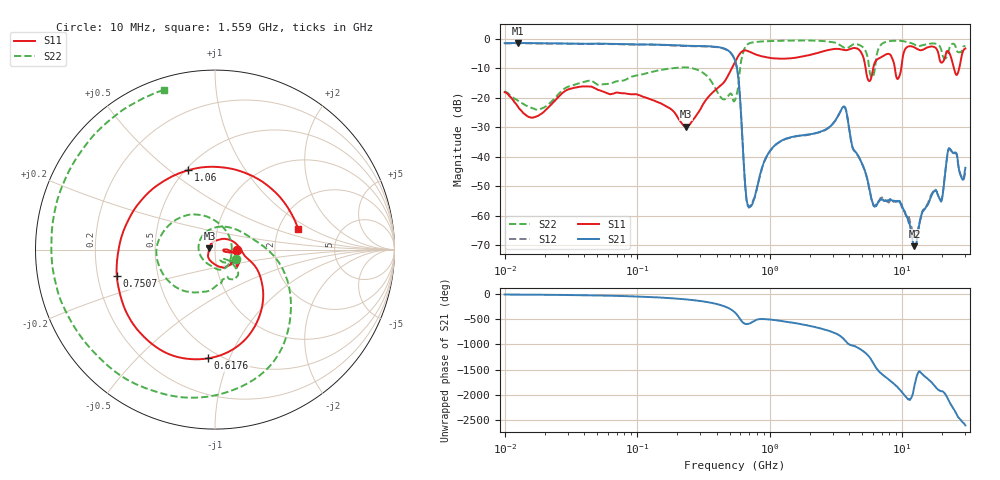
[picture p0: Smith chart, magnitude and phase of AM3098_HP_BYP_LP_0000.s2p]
!Agilent Technologies,E8364B,MY43040894,A.07.50.67
!Agilent E8364B: A.07.50.67
!Date: Wednesday, June 17, 2020 09:18:11
!Correction: S11(Full 2 Port(1,2))
!S21(Full 2 Port(1,2))
!S12(Full 2 Port(1,2))
!S22(Full 2 Port(1,2))
!S2P File: Measurements: S11, S21, S12, S22:Log Frequency Sweep
# Hz S  dB  R 50
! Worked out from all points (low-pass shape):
!   1601 points, 10 MHz to 30 GHz, reference 50 ohm
!   highest |S21| = -1.43 dB at 12.59 MHz (marker M1); lowest = -70.3 dB at 12.37 GHz (marker M2)
!   |S21| within 3 dB of the highest: start of sweep to 500.4 MHz
!   lowest |S11| = -29.8 dB at 235.1 MHz (marker M3), VSWR 1.07, Z = 47 + j0.748 ohm
!   |S11| at or under -10 dB: 5.299 GHz to 6.04 GHz (741.2 MHz wide, 13.1 % of centre); 8.812 GHz to 9.845 GHz (1.033 GHz wide, 11.1 % of centre); 24.62 GHz to 26.94 GHz (2.325 GHz wide, 9.02 % of centre)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
!   |S22| runs from -24.0 to -0.6 dB; largest |S21 - S12| = 0.015
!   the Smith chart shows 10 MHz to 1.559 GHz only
!   S11 on the Smith chart (normalised r, x): 10 MHz: 1.28, -0.01; 617.6 MHz: 0.44, -0.84; 750.7 MHz: 0.28, -0.12; 1.06 GHz: 0.51, +0.58; 1.559 GHz: 2.56, +0.76
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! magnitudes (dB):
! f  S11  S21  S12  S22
! 10 MHz  -18.1  -1.5  -1.6  -17.9
! 12.59 MHz  -23.0  -1.4  -1.5  -21.0
! 38.04 MHz  -16.2  -1.7  -1.7  -14.9
! 144.7 MHz  -21.6  -2.0  -2.1  -10.7
! 235.1 MHz  -29.8  -2.3  -2.4  -9.7
! 547.7 MHz  -7.9  -7.3  -7.4  -20.8
! 617.6 MHz  -4.3  -31.0  -31.2  -6.3
! 675.8 MHz  -4.1  -55.5  -55.8  -2.0
! 750.7 MHz  -4.9  -55.2  -54.8  -1.2
! 1.06 GHz  -6.6  -36.7  -36.8  -0.7
! 1.559 GHz  -6.4  -33.1  -33.1  -0.6
! 2.084 GHz  -5.3  -32.3  -32.3  -0.6
! 3.649 GHz  -3.8  -22.9  -23.1  -3.1
! 6.049 GHz  -9.8  -56.3  -56.1  -12.6
! 7.926 GHz  -5.1  -54.9  -55.6  -0.8
! 9.302 GHz  -13.6  -55.1  -55.2  -0.7
! 12.37 GHz  -2.9  -70.3  -66.0  -1.9
! 16.96 GHz  -2.6  -52.5  -52.2  -1.6
! 19.7 GHz  -8.1  -55.2  -54.8  -3.7
! 22.67 GHz  -4.8  -37.2  -37.3  -3.3
! 25.82 GHz  -12.3  -39.1  -39.4  -4.1
! 30 GHz  -3.3  -43.7  -45.0  -2.6
